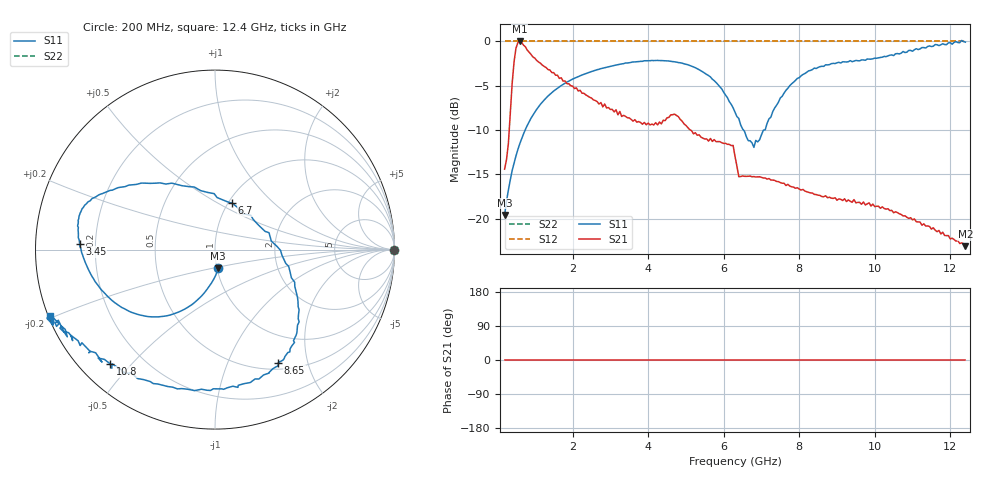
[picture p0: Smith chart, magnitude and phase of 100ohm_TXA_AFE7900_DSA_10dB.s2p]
# hz S db R 100
! AFE7900 - TX Channel A, DSA = 10dB, Fs = 11.79648 GHz
! 4/8/20
! Port 1 - SE representation of DAC differential output
! Port 2 - DAC analogoutput
! freq  dbS11  angS11
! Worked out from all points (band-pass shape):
!   245 points, 200 MHz to 12.4 GHz, reference 100 ohm
!   highest |S21| = 0.02 dB at 600 MHz (marker M1); lowest = -23.1 dB at 12.4 GHz (marker M2)
!   |S21| within 3 dB of the highest: 436.5 MHz to 1.305 GHz (868 MHz wide, 99.7 % of centre)
!   lowest |S11| = -19.6 dB at 200 MHz (marker M3), VSWR 1.23, Z = 101 - j21.2 ohm
!   |S11| at or under -10 dB: start of sweep to 744 MHz; 6.526 GHz to 7.072 GHz (546.7 MHz wide, 8.04 % of centre)
!   |S22| runs from 0.0 to 0.0 dB; largest |S21 - S12| = 0.93
!   S11 on the Smith chart (normalised r, x): 200 MHz: 1.01, -0.21; 3.45 GHz: 0.14, +0.02; 6.7 GHz: 1.04, +0.58; 8.65 GHz: 0.59, -1.54; 10.8 GHz: 0.09, -0.44; 12.4 GHz: 0.01, -0.19
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2e8  -19.57 -80.9  -14.41 0.0  0.00 0.0  0.00 0.0
3e8  -16.77 -88.8  -11.52 0.0  0.00 0.0  0.00 0.0
4.5e8  -13.73 -98.8  -2.33 0.0  0.00 0.0  0.00 0.0
6e8  -11.57 -105.6  0.02 0.0  0.00 0.0  0.00 0.0
1.35e9  -6.17 -130.3  -3.18 0.0  0.00 0.0  0.00 0.0
2.25e9  -3.80 -155.0  -5.85 0.0  0.00 0.0  0.00 0.0
3.45e9  -2.44 177.7  -8.61 0.0  0.00 0.0  0.00 0.0
4.3e9  -2.17 165.6  -9.10 0.0  0.00 0.0  0.00 0.0
4.7e9  -2.31 161.1  -8.21 0.0  0.00 0.0  0.00 0.0
5.35e9  -3.20 152.7  -10.54 0.0  0.00 0.0  0.00 0.0
6.3e9  -7.97 117.1  -12.96 0.0  0.00 0.0  0.00 0.0
6.4e9  -8.69 108.4  -15.25 0.0  0.00 0.0  0.00 0.0
6.7e9  -11.21 69.7  -15.19 0.0  0.00 0.0  0.00 0.0
6.95e9  -11.10 29.1  -15.26 0.0  0.00 0.0  0.00 0.0
7.5e9  -6.39 -22.2  -15.92 0.0  0.00 0.0  0.00 0.0
8.35e9  -3.19 -52.8  -17.10 0.0  0.00 0.0  0.00 0.0
8.65e9  -2.83 -60.8  -17.52 0.0  0.00 0.0  0.00 0.0
9.5e9  -2.16 -86.5  -18.20 0.0  0.00 0.0  0.00 0.0
1.04e10  -1.57 -120.3  -19.08 0.0  0.00 0.0  0.00 0.0
1.08e10  -1.27 -132.5  -19.66 0.0  0.00 0.0  0.00 0.0
1.14e10  -0.59 -149.3  -20.80 0.0  0.00 0.0  0.00 0.0
1.24e10  -0.10 -158.0  -23.08 0.0  0.00 0.0  0.00 0.0
